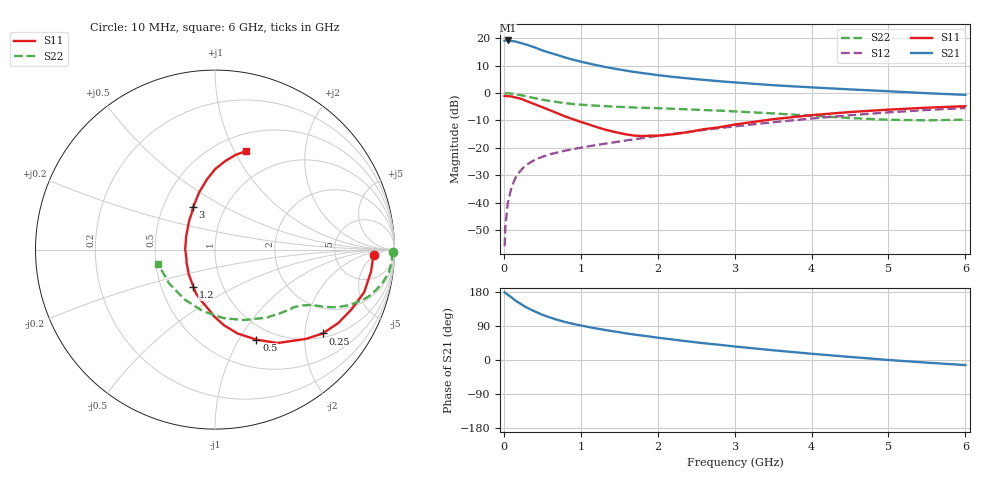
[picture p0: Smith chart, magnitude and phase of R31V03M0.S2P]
! SIEMENS Small Signal Semiconductors
! BFR181
! Si NPN RF Bipolar Junction Transistor in SOT23
! VCE = 1 V  IC = 3 mA
! Common Emitter S-Parameters:  May  1996
# GHz  S  MA  R  50
!  f  S11  S21  S12  S22
! GHz  MAG  ANG  MAG  ANG  MAG  ANG  MAG  ANG
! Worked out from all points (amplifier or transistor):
!   36 points, 10 MHz to 6 GHz, reference 50 ohm
!   highest |S21| = 19.2 dB at 50 MHz (marker M1)
!   |S21| within 3 dB of that: start of sweep to 443.2 MHz
!   unconditionally stable (mu >= 1): 1.261 GHz to 3.355 GHz
!   at 250 MHz: K = 0.31, MSG = 22.7 dB, |S12| = -27.3 dB
!   at 1.4 GHz: K = 1.04, MAG = 12.4 dB, |S12| = -18.1 dB
!   at 6 GHz: K = 0.89, MSG = 2.4 dB, |S12| = -5.5 dB
!   S11 on the Smith chart (normalised r, x): 10 MHz: 16, -4; 250 MHz: 1.11, -2.47; 500 MHz: 0.82, -1.19; 1.2 GHz: 0.73, -0.32; 3 GHz: 0.71, +0.36; 6 GHz: 0.68, +1.11
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0.01  0.8879 -1.8  9.021 178.7  0.0016 85.5  0.9934 -0.8
0.02  0.8814 -3.4  9.071 176.8  0.0036 92.1  0.9877 -1.6
0.05  0.8779 -8.1  9.117 172.4  0.0095 86.0  0.9871 -3.8
0.1  0.8641 -16.0  8.881 165.2  0.0191 80.0  0.9768 -7.5
0.15  0.8305 -23.6  8.725 156.9  0.028 76.0  0.9526 -11.1
0.25  0.7608 -37.9  7.958 144.1  0.0431 69.4  0.8978 -16.7
0.3  0.7091 -44.6  7.601 138.0  0.0496 66.7  0.8665 -19.1
0.4  0.6258 -56.3  6.82 128.4  0.0601 62.4  0.8071 -22.6
0.5  0.5518 -65.3  6.003 119.4  0.0685 59.5  0.757 -25.0
0.6  0.4846 -74.9  5.423 112.2  0.0763 57.6  0.7161 -26.6
0.7  0.4253 -83.1  4.922 105.7  0.0825 56.6  0.6812 -27.8
0.8  0.3725 -90.7  4.44 100.2  0.0888 55.8  0.6528 -28.7
0.9  0.3319 -96.6  4.053 95.3  0.0947 55.7  0.6305 -29.4
1.1  0.268 -113.0  3.479 87.1  0.1064 55.8  0.5997 -31.1
1.2  0.2406 -120.0  3.242 83.2  0.1122 56.0  0.5875 -31.9
1.6  0.1749 -155.0  2.545 69.9  0.137 57.0  0.5524 -35.2
2.2  0.1769 155.0  1.969 53.9  0.1798 57.1  0.515 -42.4
3  0.266 117.2  1.563 35.7  0.2463 54.0  0.4617 -55.8
3.5  0.3327 105.2  1.39 25.7  0.2933 50.4  0.4245 -67.7
4.5  0.45 89.7  1.166 8.1  0.3931 40.5  0.3498 -101.1
5.5  0.5403 77.7  0.992 -7.0  0.4897 27.7  0.3178 -143.7
6  0.5753 72.6  0.926 -13.4  0.5322 20.6  0.326 -165.5
